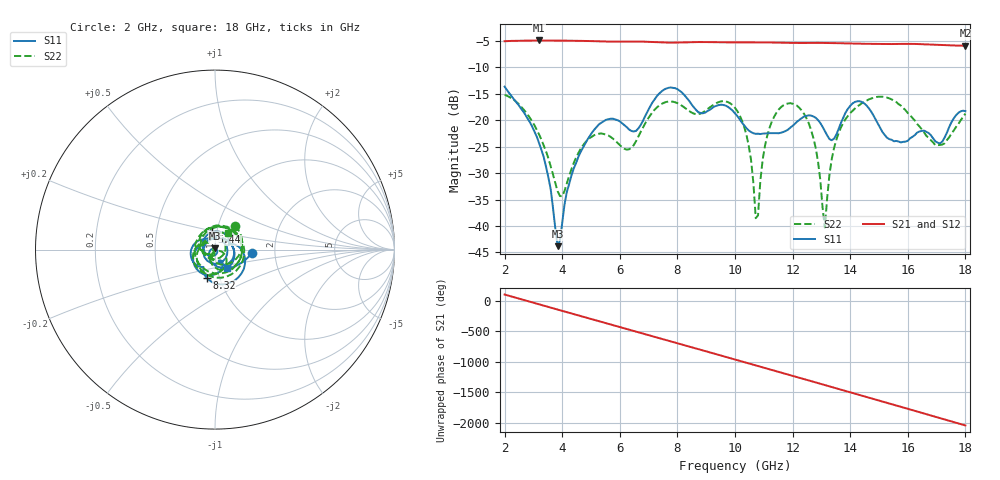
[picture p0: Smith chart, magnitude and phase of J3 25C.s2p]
!Agilent Technologies,E8363B,SG43030131,A.07.50.48
!Agilent E8363B: A.07.50.48
!Date: Wednesday, December 17, 2025 22:18:08
!Correction: S11(Full 2 Port(1,2))
!S21(Full 2 Port(1,2))
!S12(Full 2 Port(1,2))
!S22(Full 2 Port(1,2))
!S2P File: Measurements: S11, S21, S12, S22:
# Hz S  dB  R 50
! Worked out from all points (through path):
!   201 points, 2 GHz to 18 GHz, reference 50 ohm
!   highest |S21| = -4.91 dB at 3.2 GHz (marker M1); lowest = -5.9 dB at 18 GHz (marker M2)
!   group delay of S21, straight-line fit = 372 ps
!   lowest |S11| = -43.8 dB at 3.84 GHz (marker M3), VSWR 1.01, Z = 50.1 + j0.638 ohm
!   |S11| at or under -10 dB: start of sweep to end of sweep
!   |S22| runs from -40.3 to -15.2 dB; largest |S21 - S12| = 0.0012
!   S11 on the Smith chart (normalised r, x): 2 GHz: 1.52, -0.06; 5.44 GHz: 0.95, +0.18; 8.32 GHz: 0.87, -0.28; 18 GHz: 1.12, -0.23
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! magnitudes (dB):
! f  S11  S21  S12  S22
! 2 GHz  -13.7  -5.1  -5.0  -15.2
! 3.2 GHz  -24.4  -4.9  -4.9  -22.7
! 3.84 GHz  -43.8  -4.9  -4.9  -33.4
! 4.72 GHz  -25.2  -5.0  -5.0  -24.8
! 5.44 GHz  -20.2  -5.1  -5.1  -22.6
! 6.32 GHz  -21.8  -5.1  -5.1  -25.5
! 7.36 GHz  -15.0  -5.3  -5.3  -17.2
! 8.32 GHz  -15.7  -5.3  -5.3  -17.9
! 10 GHz  -18.7  -5.3  -5.3  -17.7
! 10.48 GHz  -22.0  -5.3  -5.3  -24.9
! 10.72 GHz  -22.6  -5.3  -5.3  -38.5
! 11.04 GHz  -22.5  -5.3  -5.3  -24.9
! 11.44 GHz  -22.4  -5.3  -5.3  -18.6
! 12.16 GHz  -20.3  -5.4  -5.4  -17.3
! 12.72 GHz  -19.3  -5.4  -5.4  -23.3
! 13.12 GHz  -22.1  -5.4  -5.4  -40.3
! 13.36 GHz  -23.8  -5.4  -5.4  -27.3
! 13.76 GHz  -19.5  -5.4  -5.4  -20.5
! 14.4 GHz  -16.5  -5.5  -5.5  -16.8
! 15.36 GHz  -23.6  -5.6  -5.6  -15.9
! 16.96 GHz  -24.0  -5.7  -5.7  -24.7
! 18 GHz  -18.3  -5.9  -5.9  -18.7
